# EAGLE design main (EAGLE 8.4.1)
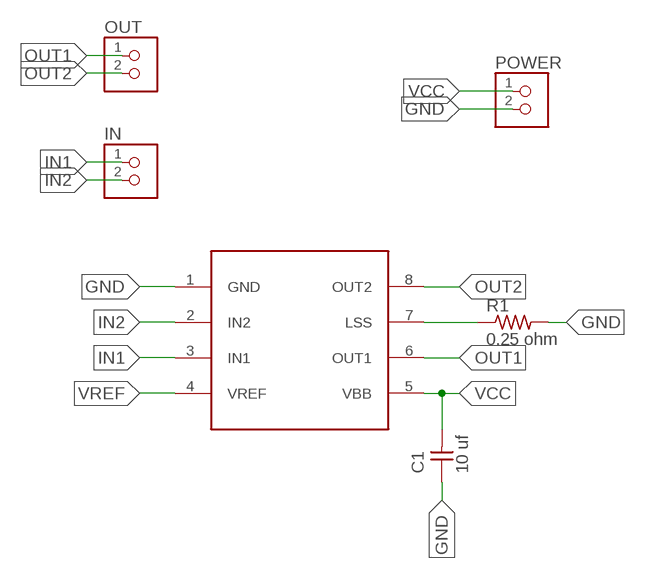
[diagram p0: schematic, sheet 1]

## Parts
C1  10 uf  CAP-UNPOLARIZEDFAB  [C1206FAB]
IN  TERM-1X02-FABLAB  [ED555DS-2DS]
OUT  TERM-1X02-FABLAB  [ED555DS-2DS]
POWER  TERM-1X02-FABLAB  [ED555DS-2DS]
R1  0.25 ohm  RES-US1206FAB  [R1206FAB]
U$1  A4953  A4953-H-BRIDGE-MOTOR-DRIVER  [SOIC8]

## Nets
GND: C1.1 POWER.2 R1.2 U$1.1(GND)
IN1: IN.1 U$1.3(IN1)
IN2: IN.2 U$1.2(IN2)
N$1: R1.1 U$1.7(LSS)
OUT1: OUT.1 U$1.6(OUT1)
OUT2: OUT.2 U$1.8(OUT2)
VCC: C1.2 POWER.1 U$1.5(VBB)
VREF: U$1.4(VREF)

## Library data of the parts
C1 = fab:CAP-UNPOLARIZED
IN OUT POWER = fab:TERM-1X02: 3.5mm terminal block, 2 positions ED555-2DS as found in the fablab inventory.
R1 = fab:RES-US: Resistor (US Symbol)
U$1 = fab:A4953-H-BRIDGE-MOTOR-DRIVER

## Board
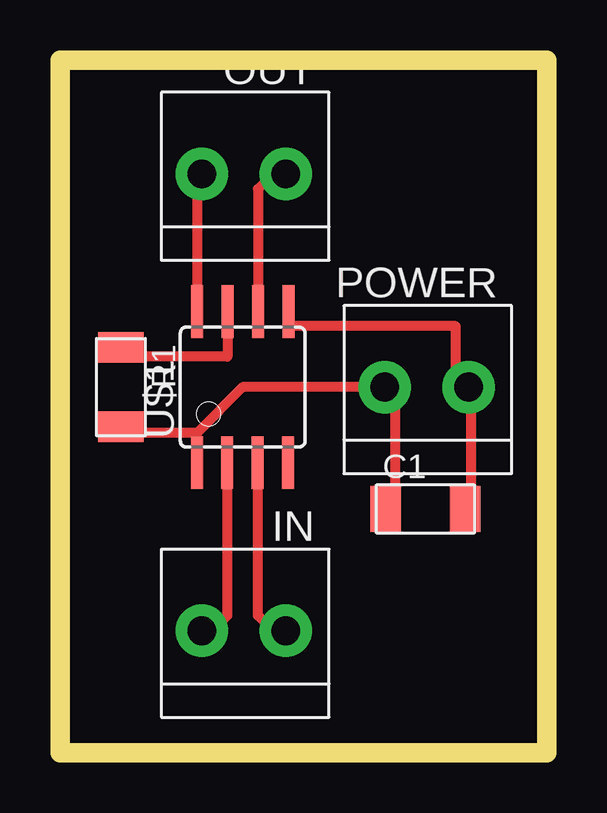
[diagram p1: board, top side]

Size 20.3 x 28.88 mm. Coordinates in mm from the lower left corner, seen from the top.
Outline: 0,0 20.3,0 20.3,28.88 0,28.88 0,0
Copper layers (1*16): Top 0.035mm / dielectric 1.5mm / Bottom 0.035mm
Design rules "default *": minimum track width 16mil, minimum drill 0.35mm, track to track 16mil, track to pad 16mil, pad to pad 16mil, via to via 16mil, smd to smd 16mil, copper to edge 16mil, drill to drill 16mil, minimum pad ring 10mil, minimum via ring 8mil, stop-mask expansion 4mil, vias tented up to drill 0mil, thermal gap 10mil

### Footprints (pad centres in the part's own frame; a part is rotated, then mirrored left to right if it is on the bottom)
C1206FAB = smd 1.27 x 1.905: 1 -1.651,0; 2 1.651,0
ED555DS-2DS = drill 1.2 pad 2.184: 1 1.8,0; 2 -1.7,0
R1206FAB = smd 1.27 x 1.905: 1 -1.651,0; 2 1.651,0
SOIC8 = smd 0.5 x 2.2: 1 -1.905,-3.154; 2 -0.645,-3.154; 3 0.625,-3.154; 4 1.895,-3.154; 5 1.905,3.154; 6 0.635,3.154; 7 -0.635,3.154; 8 -1.905,3.154

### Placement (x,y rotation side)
C1  15.24,10.16 0 top
IN  7.62,5.08 0 top
OUT  7.62,24.13 0 top
POWER  15.24,15.24 0 top
R1  2.54,15.24 270 top
U$1  7.62,15.24 0 top

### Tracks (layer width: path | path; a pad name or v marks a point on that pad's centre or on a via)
GND
  Top 0.406: 5.71,13.34 2.54,13.34 R1.2 | U$1.1 5.71,13.34 | C1.1 13.97,10.16 13.97,15.24 POWER.2 7.62,15.24 5.71,13.34
IN1
  Top 0.406: U$1.3 8.26,12.07 8.26,5.71 8.89,5.08 IN.1
IN2
  Top 0.406: U$1.2 6.98,12.07 6.98,5.71 6.35,5.08 IN.2
N$1
  Top 0.406: U$1.7 6.98,16.51 2.54,16.51 R1.1
OUT1
  Top 0.406: U$1.6 8.26,23.5 8.89,24.13 OUT.1
OUT2
  Top 0.406: U$1.8 5.71,24.13 OUT.2
VCC
  Top 0.406: C1.2 17.15,10.16 17.15,15.24 POWER.1 16.51,15.24 16.51,17.78 9.53,17.78 U$1.5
